| TEXAS INSTRUMENTS INCORPORATED
| Standard Linear and Logic Group
| IBIS Model of SN74AVC24T245
| 24-BIT DUAL-SUPPLY TRANSCIEVER WITH CONFIGURABLE VOLTAGE TRANSLATION
| AND 3-STATE OUTPUTS
| This file contains package information for the following:
|  VFBGA 83-pin (GRG) package as [Component] AVC24T245_GRG
| This device can be powered at the following Vccs:
|  1.2 volt Vcc
|  1.5 volt Vcc
|  1.8 volt Vcc
|  2.5 volt Vcc
|  3.3 volt Vcc
| This file provides unique models under the [Model Selector] for each Vcc.
| For operation at a specific Vcc, select the appropriate model after each
| [Model Selector] keyword.
[IBIS Ver]   3.2
[Comment char]  |_char
[File Name]   sn74avc24t245.ibs
[File Rev]   1.2 | x_die
[Date]   July 20, 2004
[Source]   Data created from TI-SPICE simulations at TI-SLL.
[Notes]   The following is an IBIS list for the AVC24T245.
   Please contact sllibis@ti.com with questions and
   comments concerning SLL IBIS models.
   - FILE REV HISTORY
   - 1.1 Release IBIS file on 06/24/04
   - 1.2 GRG package info revised 07/20/04
   - Power clamp data deleted as there is no power-clamp diode.
   - Due to the fact that the Device is 4.6-V Input/Output
   tolarent, the I/O models has some Non-Monotonic Warnings.
[Disclaimer] Property of Texas Instruments Incorporated.  Unauthorized
   reproduction and/or distribution is strictly prohibited.
   This product is protected under copyright law.
   Created  2004, (C) Copyright  2004, Texas Instruments
   Incorporated, All Rights Reserved
   UNLESS THERE IS A SIGNED, WRITTEN AGREEMENT TO THE
   CONTRARY, TEXAS INSTRUMENTS (TI) IS PROVIDING THE IBIS
   MODELS  AND WITHOUT ANY WARRANTY, EXPRESSED OR
   IMPLIED.  TI assumes no liability for:
   1) the accuracy of the IBIS models provided to your
   company;
   2) the proper functioning of these IBIS Models in your
   design or for any resulting applications; or
   3) infringement of patents, copyrights or intellectual
   property rights resulting from your use of these IBIS
   models.
   TI provides IBIS Models as a service to our customers.
   You and your company shall not distribute, sell or give
   these models to anyone else without prior written
   permission from TI.
   TI reserves the right to make changes to our products or
   to discontinue any semiconductor product or service
   without notice, and advises our customers to obtain the
   latest version of relevant information to verify, before
   placing orders, that the information being relied on is
   current.
   Please be aware that your receipt and use of the IBIS
   information provided shall serve as acceptance of these
   terms and conditions.  If you do not accept these terms,
   you should return or destroy the IBIS models and any
   other accompanying information immediately.
| Component AVC24T245_NMU 83-pin NMU
[Component]   AVC24T245_NMU
[Manufacturer]   Texas Instruments, Inc.
[Package]
|   typ   min   max
R_pkg   0.090e+00   0.058e+00   0.132e+00
L_pkg   2.408e-09   1.531e-09   3.517e-09
C_pkg   0.286e-13   0.191e-13   0.376e-13
[Pin]   signal_name   model_name   R_pin   L_pin   C_pin
A3   4NOE   AVC24T245_DIR   0.096e+00   2.467e-09   0.234e-13
A2   5NOE   AVC24T245_DIR   0.096e+00   2.420e-09   0.242e-13
A1   6NOE   AVC24T245_DIR   0.100e+00   2.565e-09   0.239e-13
B3   VCCB   POWER   0.130e+00   3.452e-09   0.337e-13
B2   1B2   AVC24T245_IO   0.109e+00   2.841e-09   0.315e-13
B1   1B1   AVC24T245_IO   0.087e+00   2.239e-09   0.275e-13
C3   GND   GND   0.115e+00   3.042e-09   0.372e-13
C2   1B4   AVC24T245_IO   0.099e+00   2.596e-09   0.315e-13
C1   1B3   AVC24T245_IO   0.079e+00   2.042e-09   0.270e-13
D3   VCCB   POWER   0.107e+00   2.844e-09   0.354e-13
D2   2B2   AVC24T245_IO   0.092e+00   2.415e-09   0.299e-13
D1   2B1   AVC24T245_IO   0.071e+00   1.860e-09   0.252e-13
E3   GND   GND   0.100e+00   2.684e-09   0.340e-13
E2   2B4   AVC24T245_IO   0.085e+00   2.273e-09   0.276e-13
E1   2B3   AVC24T245_IO   0.064e+00   1.672e-09   0.229e-13
F2   3B2   AVC24T245_IO   0.083e+00   2.180e-09   0.279e-13
F3   GND   GND   0.105e+00   3.001e-09   0.347e-13
F1   3B1   AVC24T245_IO   0.060e+00   1.580e-09   0.213e-13
G2   3B4   AVC24T245_IO   0.072e+00   2.043e-09   0.252e-13
G1   3B3   AVC24T245_IO   0.058e+00   1.535e-09   0.191e-13
H3   VCCB   POWER   0.083e+00   2.408e-09   0.282e-13
H1   4B1   AVC24T245_IO   0.058e+00   1.531e-09   0.191e-13
H2   4B2   AVC24T245_IO   0.072e+00   2.037e-09   0.251e-13
J1   4B3   AVC24T245_IO   0.060e+00   1.572e-09   0.212e-13
J3   GND   GND   0.105e+00   2.991e-09   0.350e-13
J2   4B4   AVC24T245_IO   0.083e+00   2.173e-09   0.279e-13
K1   5B1   AVC24T245_IO   0.064e+00   1.674e-09   0.231e-13
K2   5B2   AVC24T245_IO   0.085e+00   2.269e-09   0.277e-13
K3   GND   GND   0.101e+00   2.713e-09   0.343e-13
L1   5B3   AVC24T245_IO   0.071e+00   1.861e-09   0.255e-13
L2   5B4   AVC24T245_IO   0.091e+00   2.413e-09   0.302e-13
L3   VCCB   POWER   0.109e+00   2.911e-09   0.362e-13
M1   6B1   AVC24T245_IO   0.078e+00   2.036e-09   0.271e-13
M2   6B2   AVC24T245_IO   0.099e+00   2.599e-09   0.319e-13
M3   GND   GND   0.116e+00   3.070e-09   0.376e-13
N1   6B3   AVC24T245_IO   0.087e+00   2.235e-09   0.277e-13
N2   6B4   AVC24T245_IO   0.108e+00   2.829e-09   0.317e-13
N3   VCCB   POWER   0.131e+00   3.491e-09   0.349e-13
P1   6DIR   AVC24T245_OE   0.099e+00   2.548e-09   0.245e-13
P2   5DIR   AVC24T245_OE   0.095e+00   2.424e-09   0.252e-13
P3   4DIR   AVC24T245_OE   0.095e+00   2.458e-09   0.240e-13
P4   3DIR   AVC24T245_OE   0.095e+00   2.460e-09   0.238e-13
P5   2DIR   AVC24T245_OE   0.095e+00   2.420e-09   0.247e-13
P6   1DIR   AVC24T245_OE   0.100e+00   2.586e-09   0.247e-13
N4   VCCA   POWER   0.131e+00   3.485e-09   0.349e-13
N5   6A4   AVC24T245_IO   0.109e+00   2.831e-09   0.318e-13
N6   6A3   AVC24T245_IO   0.087e+00   2.233e-09   0.278e-13
M4   GND   GND   0.116e+00   3.069e-09   0.376e-13
M5   6A2   AVC24T245_IO   0.099e+00   2.595e-09   0.319e-13
M6   6A1   AVC24T245_IO   0.078e+00   2.034e-09   0.271e-13
L4   VCCB   POWER   0.108e+00   2.880e-09   0.360e-13
L5   5A4   AVC24T245_IO   0.091e+00   2.411e-09   0.302e-13
L6   5A3   AVC24T245_IO   0.071e+00   1.859e-09   0.255e-13
K4   GND   GND   0.101e+00   2.716e-09   0.345e-13
K5   5A2   AVC24T245_IO   0.085e+00   2.274e-09   0.279e-13
K6   5A1   AVC24T245_IO   0.064e+00   1.675e-09   0.232e-13
J5   4A4   AVC24T245_IO   0.083e+00   2.182e-09   0.282e-13
J4   GND   GND   0.105e+00   3.002e-09   0.354e-13
J6   4A3   AVC24T245_IO   0.060e+00   1.582e-09   0.215e-13
H5   4A2   AVC24T245_IO   0.081e+00   2.344e-09   0.288e-13
H6   4A1   AVC24T245_IO   0.058e+00   1.542e-09   0.194e-13
H4   VCCA   POWER   0.083e+00   2.419e-09   0.284e-13
G6   3A3   AVC24T245_IO   0.058e+00   1.546e-09   0.193e-13
G5   3A4   AVC24T245_IO   0.081e+00   2.348e-09   0.288e-13
F6   3A1   AVC24T245_IO   0.060e+00   1.591e-09   0.216e-13
F4   GND   GND   0.105e+00   3.009e-09   0.350e-13
F5   3A2   AVC24T245_IO   0.084e+00   2.194e-09   0.283e-13
E6   2A3   AVC24T245_IO   0.064e+00   1.690e-09   0.234e-13
E5   2A4   AVC24T245_IO   0.086e+00   2.289e-09   0.285e-13
E4   GND   GND   0.100e+00   2.695e-09   0.344e-13
D6   2A1   AVC24T245_IO   0.072e+00   1.877e-09   0.257e-13
D5   2A2   AVC24T245_IO   0.092e+00   2.430e-09   0.304e-13
D4   VCCA   POWER   0.108e+00   2.897e-09   0.362e-13
C6   1A3   AVC24T245_IO   0.079e+00   2.053e-09   0.274e-13
C5   1A4   AVC24T245_IO   0.100e+00   2.614e-09   0.321e-13
C4   GND   GND   0.116e+00   3.056e-09   0.376e-13
B6   1A1   AVC24T245_IO   0.087e+00   2.255e-09   0.280e-13
B5   1A2   AVC24T245_IO   0.109e+00   2.852e-09   0.313e-13
B4   VCCA   POWER   0.132e+00   3.517e-09   0.342e-13
A6   1NOE   AVC24T245_DIR   0.100e+00   2.571e-09   0.243e-13
A5   2NOE   AVC24T245_DIR   0.096e+00   2.440e-09   0.248e-13
A4   3NOE   AVC24T245_DIR   0.096e+00   2.471e-09   0.244e-13
G4   GND   GND   0.077e+00   2.843e-09   0.375e-13
| Component AVC24T245_GRG 83-pin GRG
[Component]   AVC24T245_GRG
[Manufacturer]   Texas Instruments, Inc.
[Package]
|   typ   min   max
R_pkg   0.090e+00   0.058e+00   0.132e+00
L_pkg   2.408e-09   1.531e-09   3.517e-09
C_pkg   0.286e-13   0.191e-13   0.376e-13
[Pin]   signal_name   model_name   R_pin   L_pin   C_pin
A3   4NOE   AVC24T245_DIR   0.096e+00   2.467e-09   0.234e-13
A2   5NOE   AVC24T245_DIR   0.096e+00   2.420e-09   0.242e-13
A1   6NOE   AVC24T245_DIR   0.100e+00   2.565e-09   0.239e-13
B3   VCCB   POWER   0.130e+00   3.452e-09   0.337e-13
B2   1B2   AVC24T245_IO   0.109e+00   2.841e-09   0.315e-13
B1   1B1   AVC24T245_IO   0.087e+00   2.239e-09   0.275e-13
C3   GND   GND   0.115e+00   3.042e-09   0.372e-13
C2   1B4   AVC24T245_IO   0.099e+00   2.596e-09   0.315e-13
C1   1B3   AVC24T245_IO   0.079e+00   2.042e-09   0.270e-13
D3   VCCB   POWER   0.107e+00   2.844e-09   0.354e-13
D2   2B2   AVC24T245_IO   0.092e+00   2.415e-09   0.299e-13
D1   2B1   AVC24T245_IO   0.071e+00   1.860e-09   0.252e-13
E3   GND   GND   0.100e+00   2.684e-09   0.340e-13
E2   2B4   AVC24T245_IO   0.085e+00   2.273e-09   0.276e-13
E1   2B3   AVC24T245_IO   0.064e+00   1.672e-09   0.229e-13
F2   3B2   AVC24T245_IO   0.083e+00   2.180e-09   0.279e-13
F3   GND   GND   0.105e+00   3.001e-09   0.347e-13
F1   3B1   AVC24T245_IO   0.060e+00   1.580e-09   0.213e-13
G2   3B4   AVC24T245_IO   0.072e+00   2.043e-09   0.252e-13
G1   3B3   AVC24T245_IO   0.058e+00   1.535e-09   0.191e-13
H3   VCCB   POWER   0.083e+00   2.408e-09   0.282e-13
H1   4B1   AVC24T245_IO   0.058e+00   1.531e-09   0.191e-13
H2   4B2   AVC24T245_IO   0.072e+00   2.037e-09   0.251e-13
J1   4B3   AVC24T245_IO   0.060e+00   1.572e-09   0.212e-13
J3   GND   GND   0.105e+00   2.991e-09   0.350e-13
J2   4B4   AVC24T245_IO   0.083e+00   2.173e-09   0.279e-13
K1   5B1   AVC24T245_IO   0.064e+00   1.674e-09   0.231e-13
K2   5B2   AVC24T245_IO   0.085e+00   2.269e-09   0.277e-13
K3   GND   GND   0.101e+00   2.713e-09   0.343e-13
L1   5B3   AVC24T245_IO   0.071e+00   1.861e-09   0.255e-13
L2   5B4   AVC24T245_IO   0.091e+00   2.413e-09   0.302e-13
L3   VCCB   POWER   0.109e+00   2.911e-09   0.362e-13
M1   6B1   AVC24T245_IO   0.078e+00   2.036e-09   0.271e-13
M2   6B2   AVC24T245_IO   0.099e+00   2.599e-09   0.319e-13
M3   GND   GND   0.116e+00   3.070e-09   0.376e-13
N1   6B3   AVC24T245_IO   0.087e+00   2.235e-09   0.277e-13
N2   6B4   AVC24T245_IO   0.108e+00   2.829e-09   0.317e-13
N3   VCCB   POWER   0.131e+00   3.491e-09   0.349e-13
P1   6DIR   AVC24T245_OE   0.099e+00   2.548e-09   0.245e-13
P2   5DIR   AVC24T245_OE   0.095e+00   2.424e-09   0.252e-13
P3   4DIR   AVC24T245_OE   0.095e+00   2.458e-09   0.240e-13
P4   3DIR   AVC24T245_OE   0.095e+00   2.460e-09   0.238e-13
P5   2DIR   AVC24T245_OE   0.095e+00   2.420e-09   0.247e-13
P6   1DIR   AVC24T245_OE   0.100e+00   2.586e-09   0.247e-13
N4   VCCA   POWER   0.131e+00   3.485e-09   0.349e-13
N5   6A4   AVC24T245_IO   0.109e+00   2.831e-09   0.318e-13
N6   6A3   AVC24T245_IO   0.087e+00   2.233e-09   0.278e-13
M4   GND   GND   0.116e+00   3.069e-09   0.376e-13
M5   6A2   AVC24T245_IO   0.099e+00   2.595e-09   0.319e-13
M6   6A1   AVC24T245_IO   0.078e+00   2.034e-09   0.271e-13
L4   VCCB   POWER   0.108e+00   2.880e-09   0.360e-13
L5   5A4   AVC24T245_IO   0.091e+00   2.411e-09   0.302e-13
L6   5A3   AVC24T245_IO   0.071e+00   1.859e-09   0.255e-13
K4   GND   GND   0.101e+00   2.716e-09   0.345e-13
K5   5A2   AVC24T245_IO   0.085e+00   2.274e-09   0.279e-13
K6   5A1   AVC24T245_IO   0.064e+00   1.675e-09   0.232e-13
J5   4A4   AVC24T245_IO   0.083e+00   2.182e-09   0.282e-13
J4   GND   GND   0.105e+00   3.002e-09   0.354e-13
J6   4A3   AVC24T245_IO   0.060e+00   1.582e-09   0.215e-13
H5   4A2   AVC24T245_IO   0.081e+00   2.344e-09   0.288e-13
H6   4A1   AVC24T245_IO   0.058e+00   1.542e-09   0.194e-13
H4   VCCA   POWER   0.083e+00   2.419e-09   0.284e-13
G6   3A3   AVC24T245_IO   0.058e+00   1.546e-09   0.193e-13
G5   3A4   AVC24T245_IO   0.081e+00   2.348e-09   0.288e-13
F6   3A1   AVC24T245_IO   0.060e+00   1.591e-09   0.216e-13
F4   GND   GND   0.105e+00   3.009e-09   0.350e-13
F5   3A2   AVC24T245_IO   0.084e+00   2.194e-09   0.283e-13
E6   2A3   AVC24T245_IO   0.064e+00   1.690e-09   0.234e-13
E5   2A4   AVC24T245_IO   0.086e+00   2.289e-09   0.285e-13
E4   GND   GND   0.100e+00   2.695e-09   0.344e-13
D6   2A1   AVC24T245_IO   0.072e+00   1.877e-09   0.257e-13
D5   2A2   AVC24T245_IO   0.092e+00   2.430e-09   0.304e-13
D4   VCCA   POWER   0.108e+00   2.897e-09   0.362e-13
C6   1A3   AVC24T245_IO   0.079e+00   2.053e-09   0.274e-13
C5   1A4   AVC24T245_IO   0.100e+00   2.614e-09   0.321e-13
C4   GND   GND   0.116e+00   3.056e-09   0.376e-13
B6   1A1   AVC24T245_IO   0.087e+00   2.255e-09   0.280e-13
B5   1A2   AVC24T245_IO   0.109e+00   2.852e-09   0.313e-13
B4   VCCA   POWER   0.132e+00   3.517e-09   0.342e-13
A6   1NOE   AVC24T245_DIR   0.100e+00   2.571e-09   0.243e-13
A5   2NOE   AVC24T245_DIR   0.096e+00   2.440e-09   0.248e-13
A4   3NOE   AVC24T245_DIR   0.096e+00   2.471e-09   0.244e-13
G4   GND   GND   0.077e+00   2.843e-09   0.375e-13
| Model AVC24T245_DIR
[Model Selector]   AVC24T245_DIR
AVC24T245_DIR_12   1.2 volt Vcc
AVC24T245_DIR_15   1.5 volt Vcc
AVC24T245_DIR_18   1.8 volt Vcc
AVC24T245_DIR_25   2.5 volt Vcc
AVC24T245_DIR_33   3.3 volt Vcc
| Model AVC24T245_OE
[Model Selector]   AVC24T245_OE
AVC24T245_OE_12   1.2 volt Vcc
AVC24T245_OE_15   1.5 volt Vcc
AVC24T245_OE_18   1.8 volt Vcc
AVC24T245_OE_25   2.5 volt Vcc
AVC24T245_OE_33   3.3 volt Vcc
| Model AVC24T245_IO
[Model Selector]   AVC24T245_IO
AVC24T245_IO_12   1.2 volt Vcc
AVC24T245_IO_15   1.5 volt Vcc
AVC24T245_IO_18   1.8 volt Vcc
AVC24T245_IO_25   2.5 volt Vcc
AVC24T245_IO_33   3.3 volt Vcc
| Models and submodels in the file (15): AVC24T245_DIR_12 (Input), AVC24T245_DIR_15 (Input), AVC24T245_DIR_18 (Input), AVC24T245_DIR_25 (Input), AVC24T245_DIR_33 (Input), AVC24T245_OE_12 (Input), AVC24T245_OE_15 (Input), AVC24T245_OE_18 (Input), AVC24T245_OE_25 (Input), AVC24T245_OE_33 (Input), AVC24T245_IO_12 (I/O), AVC24T245_IO_15 (I/O), AVC24T245_IO_18 (I/O), AVC24T245_IO_25 (I/O), AVC24T245_IO_33 (I/O)
